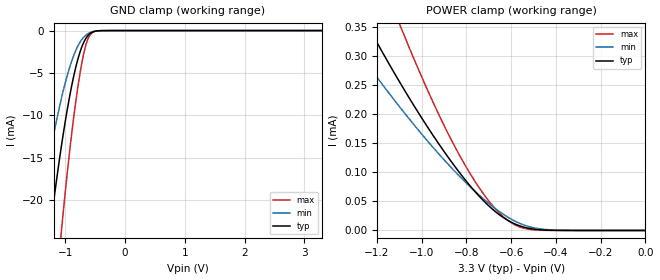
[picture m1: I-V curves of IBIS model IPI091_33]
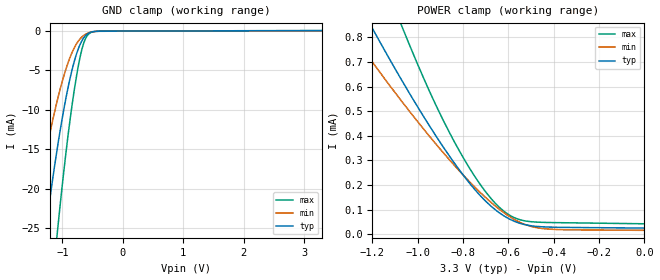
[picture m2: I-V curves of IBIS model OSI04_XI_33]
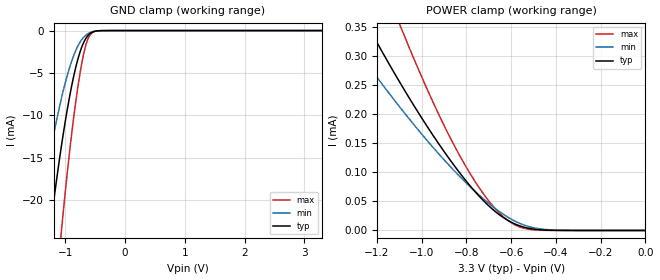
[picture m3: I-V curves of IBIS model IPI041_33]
| TEXAS INSTRUMENTS INCORPORATED
| Connectivity Solutions Group
| IBIS Model of UART2550_33V
| UART2550_33V
| This file contains package information for the following:
|  PFB 48-pin (PQFP) package as [Component] UART2550_33V_PQFP
| This device can be powered at the following Vccs:
|  3.3 volt Vcc
| This file provides unique models under the [Model Selector] for each Vcc.
| For operation at a specific Vcc, select the appropriate model after each
| [Model Selector] keyword.
[IBIS Ver]   3.2
[Comment char]  |_char
[File Name]   uart2550_33v.ibs
[File Rev]   1 | a
[Date]   November 10, 2003
[Source]   Data created from TI-SPICE simulations at TI-CONN.
[Notes]   The following is an IBIS list for the UART2550_33V.
   Please contact s-ly@ti.com with questions and
   comments concerning CONN IBIS models.
[Disclaimer] Property of Texas Instruments Incorporated.  Unauthorized
   reproduction and/or distribution is strictly prohibited.
   This product is protected under copyright law.
   Created  2003, (C) Copyright  2003, Texas Instruments
   Incorporated, All Rights Reserved
   UNLESS THERE IS A SIGNED, WRITTEN AGREEMENT TO THE
   CONTRARY, TEXAS INSTRUMENTS (TI) IS PROVIDING THE IBIS
   MODELS  AND WITHOUT ANY WARRANTY, EXPRESSED OR
   IMPLIED.  TI assumes no liability for:
   1) the accuracy of the IBIS models provided to your
   company;
   2) the proper functioning of these IBIS Models in your
   design or for any resulting applications; or
   3) infringement of patents, copyrights or intellectual
   property rights resulting from your use of these IBIS
   models.
   TI provides IBIS Models as a service to our customers.
   You and your company shall not distribute, sell or give
   these models to anyone else without prior written
   permission from TI.
   TI reserves the right to make changes to our products or
   to discontinue any semiconductor product or service
   without notice, and advises our customers to obtain the
   latest version of relevant information to verify, before
   placing orders, that the information being relied on is
   current.
   Please be aware that your receipt and use of the IBIS
   information provided shall serve as acceptance of these
   terms and conditions.  If you do not accept these terms,
   you should return or destroy the IBIS models and any
   other accompanying information immediately.
| Component UART2550_33V_PQFP 48-pin PFB
[Component]   UART2550_33V_PQFP
[Manufacturer]   Texas Instruments, Inc.
[Package]
|   typ   min   max
R_pkg   1.000e-03   1.000e-03   2.000e-03
L_pkg   1.068e-09   1.000e-09   1.094e-09
C_pkg   1.970e-13   1.710e-13   2.150e-13
[Pin]   signal_name   model_name   R_pin   L_pin   C_pin
1   D5   IPI04_OPJ43   1.000e-03   1.084e-09   1.750e-13
2   D6   IPI04_OPJ43   1.000e-03   1.087e-09   2.100e-13
3   D7   IPI04_OPJ43   2.000e-03   1.094e-09   2.140e-13
4   RXB   IPI041   2.000e-03   1.088e-09   2.110e-13
5   RXA   IPI041   2.000e-03   1.058e-09   2.000e-13
6   TXRDYB   OPJ430   1.000e-03   1.002e-09   1.710e-13
7   TXA   OPJ430   1.000e-03   1.002e-09   1.710e-13
8   TXB   OPJ430   2.000e-03   1.058e-09   2.000e-13
9   OPB   OPJ430   2.000e-03   1.088e-09   2.110e-13
10   CSA   IPI041   2.000e-03   1.094e-09   2.140e-13
11   CSB   IPI041   1.000e-03   1.087e-09   2.100e-13
12   NC   NC   1.000e-03   1.084e-09   1.750e-13
13   XTAL1   OSI04_XI   1.000e-03   1.083e-09   1.750e-13
14   XTAL2   OSI04   1.000e-03   1.085e-09   2.110e-13
15   IOW   IPI041   2.000e-03   1.093e-09   2.140e-13
16   CDB   IPI041   2.000e-03   1.087e-09   2.120e-13
17   GND   GND   2.000e-03   1.056e-09   2.000e-13
18   RXRDYB   OPJ430   1.000e-03   1.001e-09   1.710e-13
19   IOR   IPI041   1.000e-03   1.001e-09   1.710e-13
20   DSRB   IPI041   2.000e-03   1.056e-09   2.000e-13
21   RIB   IPI041   2.000e-03   1.087e-09   2.120e-13
22   RTSB   OPJ430   2.000e-03   1.093e-09   2.140e-13
23   CTSB   IPI041   1.000e-03   1.085e-09   2.110e-13
24   NC   NC   1.000e-03   1.083e-09   1.750e-13
25   NC   NC   1.000e-03   1.084e-09   1.750e-13
26   A2   IPI041   1.000e-03   1.086e-09   2.100e-13
27   A1   IPI041   2.000e-03   1.094e-09   2.140e-13
28   A0   IPI041   2.000e-03   1.088e-09   2.120e-13
29   INTB   OPJ430   2.000e-03   1.058e-09   2.000e-13
30   INTA   OPJ430   1.000e-03   1.002e-09   1.710e-13
31   RXRDYA   OPJ430   1.000e-03   1.002e-09   1.710e-13
32   OPA   OPJ430   2.000e-03   1.058e-09   2.000e-13
33   RTSA   OPJ430   2.000e-03   1.088e-09   2.120e-13
34   DTRA   OPJ430   2.000e-03   1.094e-09   2.140e-13
35   DTRB   OPJ430   1.000e-03   1.086e-09   2.100e-13
36   RESET   IPI091   1.000e-03   1.084e-09   1.750e-13
37   NC   NC   1.000e-03   1.081e-09   1.760e-13
38   CTSA   IPI041   1.000e-03   1.083e-09   2.110e-13
39   DSRA   IPI041   2.000e-03   1.091e-09   2.150e-13
40   CDA   IPI041   2.000e-03   1.085e-09   2.120e-13
41   RIA   IPI041   1.000e-03   1.055e-09   2.010e-13
42   VCC   POWER   1.000e-03   1.000e-09   1.710e-13
43   TXRDYA   OPJ430   1.000e-03   1.000e-09   1.710e-13
44   D0   IPI04_OPJ43   1.000e-03   1.055e-09   2.010e-13
45   D1   IPI04_OPJ43   2.000e-03   1.085e-09   2.120e-13
46   D2   IPI04_OPJ43   2.000e-03   1.091e-09   2.150e-13
47   D3   IPI04_OPJ43   1.000e-03   1.083e-09   2.110e-13
48   D4   IPI04_OPJ43   1.000e-03   1.081e-09   1.760e-13
| Model IPI091
[Model Selector]   IPI091
IPI091_33   3.3 volt Vcc
| Model OSI04_XI
[Model Selector]   OSI04_XI
OSI04_XI_33   3.3 volt Vcc
| Model IPI041
[Model Selector]   IPI041
IPI041_33   3.3 volt Vcc
| Model IPI04_OPJ43
[Model Selector]   IPI04_OPJ43
IPI04_OPJ43_33   3.3 volt Vcc
| Model OPJ430
[Model Selector]   OPJ430
OPJ430_33   3.3 volt Vcc
| Model OSI04
[Model Selector]   OSI04
OSI04_33   3.3 volt Vcc
| Models and submodels in the file (6): IPI091_33 (Input), OSI04_XI_33 (Input), IPI041_33 (Input), IPI04_OPJ43_33 (I/O), OPJ430_33 (3-state), OSI04_33 (3-state)
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[Model]   IPI091_33
Model_type  Input
Vinl = 0
Vinh = 3.3
| variable   typ   min   max
C_comp   1.07pF   0.95pF   1.20pF
[Temperature Range]   40   125   -40
| Ambient temperature   25   110   -40
[Voltage range]   3.3   3   3.6
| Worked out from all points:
|   GND clamp passes 1 mA (typ) near -0.66 V on its own axis
|   POWER clamp passes 1 mA (typ) near -2.03 V on its own axis
[GND Clamp]
| IPI091_33
|   Voltage   I(typ)   I(min)   I(max)
-3.3V     -184.1mA   -131.7mA   -253.5mA
-1.485V   -37.43mA   -23.94mA   -59.12mA
-1.28V    -24.78mA   -15.34mA   -40.66mA
-1.25V    -23.07mA   -14.2mA    -38.11mA
-1.075V   -13.97mA   -8.224mA   -24.19mA
-1.06V    -13.26mA   -7.774mA   -23.08mA
-940mV    -8.152mA   -4.58mA    -14.87mA
-805mV    -3.718mA   -2.005mA   -7.28mA
-700mV    -1.488mA   -825uA     -2.909mA
-600mV    -421.4uA   -273uA     -659.6uA
-400mV    -8.531uA   -12.92uA   -6.748uA
3.3V      251.6pA    69.15nA    65.83pA
[POWER Clamp]
| IPI091_33
|   Voltage   I(typ)   I(min)   I(max)
-3.3V     2.289mA    1.713mA    3.253mA
-1.35V    432uA      344.6uA    613.8uA
-1.225V   341.4uA    277.2uA    481uA
-1.11V    263.3uA    218.6uA    366.4uA
-1.075V   240.6uA    201.5uA    333.1uA
-930mV    152.9uA    134.7uA    205.1uA
-805mV    87.01uA    83.43uA    112uA
-700mV    42.42uA    46.59uA    50.87uA
-620mV    18.66uA    24.18uA    18.85uA
-540mV    5.375uA    9.01uA     3.55uA
-445mV    638.3nA    1.643uA    187.2nA
-47.99fV  251.6pA    2.2nA      73.1pA
[Model]   OSI04_XI_33
Model_type  Input
Vinl = 0
Vinh = 3.3
| variable   typ   min   max
C_comp   1.85pF   1.15pF   2.42pF
[Temperature Range]   40   125   -40
| Ambient temperature   25   110   -40
[Voltage range]   3.3   3   3.6
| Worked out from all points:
|   GND clamp passes 1 mA (typ) near -0.66 V on its own axis
|   POWER clamp passes 1 mA (typ) near -1.30 V on its own axis
[GND Clamp]
| OSI04_XI_33
|   Voltage   I(typ)   I(min)   I(max)
-3.3V     -187.4mA   -133.6mA   -258.6mA
-1.52V    -40.73mA   -26.12mA   -63.96mA
-1.48V    -38.05mA   -24.28mA   -60.12mA
-1.275V   -25.2mA    -15.59mA   -41.32mA
-1.095V   -15.43mA   -9.17mA    -26.46mA
-1.07V    -14.21mA   -8.387mA   -24.55mA
-935mV    -8.294mA   -4.704mA   -15.09mA
-800mV    -3.791mA   -2.104mA   -7.36mA
-695mV    -1.529mA   -912.1uA   -2.917mA
-600mV    -479.4uA   -361uA     -744.5uA
-390mV    -35.35uA   -32.95uA   -52.71uA
3.3V      25.17uA    17.8uA     39.06uA
[POWER Clamp]
| OSI04_XI_33
|   Voltage   I(typ)   I(min)   I(max)
-3.3V     5.294mA    3.984mA    7.572mA
-1.3V     1.007mA    827.6uA    1.402mA
-1.195V   827.7uA    692.7uA    1.14mA
-1.075V   632.4uA    545.1uA    855.7uA
-1.04V    577.7uA    503.5uA    776.7uA
-915mV    392.6uA    361.2uA    514.8uA
-815mV    259.4uA    256uA      336.3uA
-720mV    152.9uA    166.1uA    196.6uA
-625mV    77.8uA     91.06uA    97.45uA
-555mV    46.18uA    50.98uA    60.77uA
-455mV    30.55uA    24.01uA    48.59uA
-47.99fV  25.17uA    16.02uA    42.63uA
[Model]   IPI041_33
Model_type  Input
Vinl = 0
Vinh = 3.3
| variable   typ   min   max
C_comp   1.08pF   0.95pF   1.21pF
[Temperature Range]   40   125   -40
| Ambient temperature   25   110   -40
[Voltage range]   3.3   3   3.6
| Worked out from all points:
|   GND clamp passes 1 mA (typ) near -0.66 V on its own axis
|   POWER clamp passes 1 mA (typ) near -2.03 V on its own axis
[GND Clamp]
| IPI041_33
|   Voltage   I(typ)   I(min)   I(max)
-3.3V     -184.1mA   -131.7mA   -253.5mA
-1.485V   -37.43mA   -23.94mA   -59.12mA
-1.28V    -24.78mA   -15.34mA   -40.66mA
-1.25V    -23.07mA   -14.2mA    -38.11mA
-1.075V   -13.97mA   -8.224mA   -24.19mA
-1.06V    -13.26mA   -7.774mA   -23.08mA
-940mV    -8.152mA   -4.58mA    -14.87mA
-805mV    -3.718mA   -2.005mA   -7.28mA
-700mV    -1.488mA   -825uA     -2.909mA
-600mV    -421.4uA   -273uA     -659.6uA
-400mV    -8.531uA   -12.92uA   -6.748uA
3.3V      251.6pA    69.15nA    65.83pA
[POWER Clamp]
| IPI041_33
|   Voltage   I(typ)   I(min)   I(max)
-3.3V     2.289mA    1.713mA    3.253mA
-1.35V    432uA      344.6uA    613.8uA
-1.225V   341.4uA    277.2uA    481uA
-1.11V    263.3uA    218.6uA    366.4uA
-1.075V   240.6uA    201.5uA    333.1uA
-930mV    152.9uA    134.7uA    205.1uA
-805mV    87.01uA    83.43uA    112uA
-700mV    42.42uA    46.59uA    50.87uA
-620mV    18.66uA    24.18uA    18.85uA
-540mV    5.375uA    9.01uA     3.55uA
-445mV    638.3nA    1.643uA    187.2nA
-47.99fV  251.6pA    2.2nA      73.1pA
